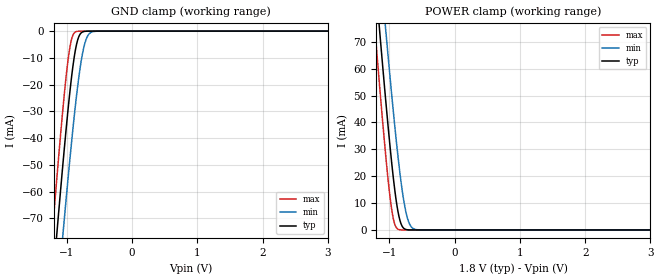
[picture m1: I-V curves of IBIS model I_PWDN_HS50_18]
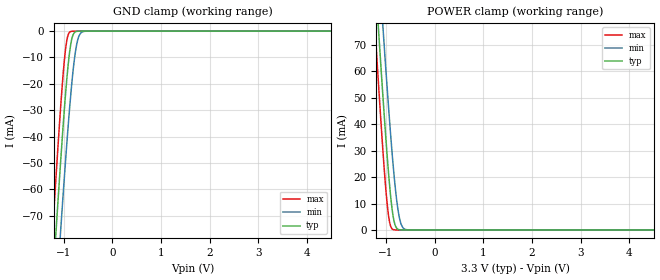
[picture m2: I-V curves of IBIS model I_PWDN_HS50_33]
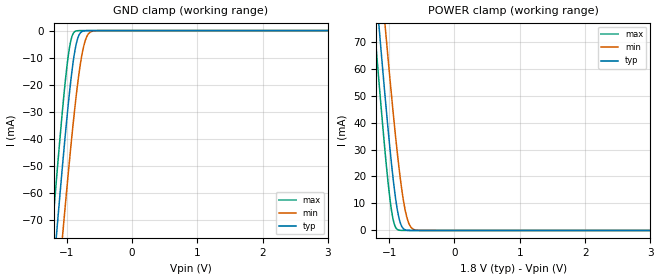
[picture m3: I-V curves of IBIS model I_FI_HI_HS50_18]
| Texas Instruments Incorporated
| DS90UB904Q
| 10-43-MHz 18-Bit Color FPD Link III Serializer and Deserializer
| with Bi-Directional Control Channel
| Marketing part#   Voltage Range   Package-type   Temperature
| DS90UB904QSQE   1.71V - 3.6V   48-Pin LLP   -40 to 105C
| DS90UB904QSQ   1.71V - 3.6V   48-Pin LLP   -40 to 105C
| DS90UB904QSQX   1.71V - 3.6V   48-Pin LLP   -40 to 105C
[IBIS Ver]   4.0
[File name]   ds90ub904q.ibs
[File Rev]   1.0
[Date]   04/11/2012
[Source]   Model built from TISPICE simulations at:
   Texas Instruments Incorporated.
   WEBENCH DESIGN CENTER
   12500 TI Blvd
   Dallas, TX -75243
   For Support e-mail: elab_scm_ibis@list.ti.com
[Notes]   Rev 1.0: 04/11/2012
   - Initial version of the IBIS model
   - All models are generated in Spectre
   - ccomp is listed in numerical order, for PVT information,
   please check notes above ccomp keyword for each model
   - All non-monotonic warnings can be ignored as per buffer behavior
[Disclaimer] This product is designed as an aid for customers of Texas Instruments.
   No warranties, either expressed or implied, with respect to this third
   party software (if any) or with respect to its fitness for any
   particular purpose is claimed by Texas Instruments or the author. The
   software (if any) is provided solely on an "as is" basis. The entire
   risk as to its quality and performance is with the customer
[Copyright]   (C)Copyright 2012 Texas Instruments Incorporated.
   All rights reserved.
|   DS90UB904Q
[Component]  DS90UB904Q
[Manufacturer]  Texas Instruments, Inc.
[Package]   |48-pin LLP 7.0x7.0x0.5mm
|   typ   min   max
R_pkg   0   0   0
L_pkg   0   0   0
C_pkg   0   0   0
[Pin]   signal_name   model_name   R_pin   L_pin   C_pin
1   SDA   IO_SMBUS_HS50
2   SCL   IO_SMBUS_HS50
3   VDDSSCG   POWER
4   PCLK   IO_CLK_50_HS50
5   ROUT[20]   IO_DATA_50_ATP_HS50
6   ROUT[19]   IO_DATA_50_HS50
7   VDDIO3   POWER
8   ROUT[18]   IO_DATA_50_HS50
9   ROUT[17]   IO_DATA_50_HS50
10   ROUT[16]   IO_DATA_50_HS50
11   ROUT[15]   IO_DATA_50_HS50
12   ROUT[14]   IO_DATA_50_HS50
13   ROUT[13]   IO_DATA_50_HS50
14   ROUT[12]   IO_DATA_50_HS50
15   ROUT[11]   IO_DATA_50_HS50
16   ROUT[10]   IO_DATA_50_HS50
17   VDDD   POWER
18   ROUT[9]   IO_DATA_50_HS50
19   ROUT[8]   IO_DATA_50_HS50
20   VDDIO2   POWER
21   ROUT[7]   IO_DATA_50_HS50
22   ROUT[6]   IO_DATA_50_HS50
23   ROUT[5]   IO_DATA_50_HS50
24   ROUT[4]   IO_DATA_50_HS50
25   ROUT[3]   IO_DATA_50_HS50
26   ROUT[2]   IO_DATA_50_HS50
27   ROUT[1]   IO_DATA_50_ATP_HS50
28   ROUT[0]   IO_DATA_50_ATP_HS50
29   VDDIO1   POWER
30   GPI[3]   IO_DATA_50_ATP_HS50
31   GPI[2]   IO_DATA_50_ATP_HS50
32   GPI[1]   IO_DATA_50_ATP_HS50
33   GPI[0]   IO_DATA_50_ATP_HS50
34   LOCK   IO_DATA_50_ATP_HS50
35   PDB   I_PWDN_HS50
36   VDDR   POWER
37   PASS   IO_DATA_50_HS50
38   RES   NC
39   RES   NC
40   VDDCML   POWER
41   RIN+   NC
42   RIN-   NC
43   RES   NC
44   BISTEN   I_PWDN_HS50
45   VDDPLL   POWER
46   RES   NC
47   MODE   I_FI_HI_HS50
48   ID[x]   NC
49   DAP   GND
[Package Model] llp48_ds90uh904
[Model Selector]   I_PWDN_HS50
I_PWDN_HS50_33   I_PWDN_HS50 input with VDD=3.3V
I_PWDN_HS50_18   I_PWDN_HS50 input with VDD=1.8V
[Model Selector]   I_FI_HI_HS50
I_FI_HI_HS50_33   I_FI_HI_HS50 input with VDD=3.3V
I_FI_HI_HS50_18   I_FI_HI_HS50 input with VDD=1.8V
[Model Selector]   IO_DATA_50_ATP_HS50
IO_DATA_50_ATP_HS50_33   IO_DATA_50_ATP_HS50 with VDD=3.3V
IO_DATA_50_ATP_HS50_18   IO_DATA_50_ATP_HS50 with VDD=1.8V
[Model Selector]   IO_DATA_50_HS50
IO_DATA_50_HS50_33   IO_DATA_50_HS50 with VDD=3.3V
IO_DATA_50_HS50_18   IO_DATA_50_HS50 with VDD=1.8V
[Model Selector]   IO_SMBUS_HS50
IO_SMBUS_HS50_33   IO_SMBUS_HS50 with VDD=3.3V
IO_SMBUS_HS50_18   IO_SMBUS_HS50 with VDD=1.8V
[Model Selector]   IO_CLK_50_HS50
IO_CLK_50_HS50_33   IO_CLK_50_HS50 with VDD=3.3V
IO_CLK_50_HS50_18   IO_CLK_50_HS50 with VDD=1.8V
|   Package model for DS90UB903
[Define Package Model]  llp48_ds90uh904
[Manufacturer]  Texas Instruments, Inc.
[OEM]  Texas Instruments, Inc.
[Description]  Package model with Au wires, simulation frequency of 1.4GHz
|Buildsheet# DS90UB904QSQ-03
[Number Of Pins]  48
[Pin Numbers]
49   | 49 = DAP
1   | 1 = L1
2   | 2 = L2
3   | 3 = L3
4   | 4 = L4
5   | 5 = L5
6   | 6 = L6
7   | 7 = L7
8   | 8 = L8
9   | 9 = L9
10   | 10 = L10
11   | 11 = L11
12   | 12 = L12
13   | 13 = L13
14   | 14 = L14
15   | 15 = L15
16   | 16 = L16
17   | 17 = L17
18   | 18 = L18
19   | 19 = L19
20   | 20 = L20
21   | 21 = L21
22   | 22 = L22
23   | 23 = L23
24   | 24 = L24
25   | 25 = L25
26   | 26 = L26
27   | 27 = L27
28   | 28 = L28
29   | 29 = L29
30   | 30 = L30
31   | 31 = L31
32   | 32 = L32
33   | 33 = L33
34   | 34 = L34
35   | 35 = L35
36   | 36 = L36
37   | 37 = L37
38   | 38 = L38
39   | 39 = L39
40   | 40 = L40
41   | 41 = L41
42   | 42 = L42
44   | 44 = L44
45   | 45 = L45
46   | 46 = L46
47   | 47 = L47
48   | 48 = L48
[Model Data]
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[End Model Data]
[End Package Model]
| Models and submodels in the file (12): I_PWDN_HS50_18 (Input), I_PWDN_HS50_33 (Input), I_FI_HI_HS50_18 (Input), I_FI_HI_HS50_33 (Input), IO_DATA_50_ATP_HS50_33 (I/O), IO_DATA_50_ATP_HS50_18 (I/O), IO_DATA_50_HS50_33 (I/O), IO_DATA_50_HS50_18 (I/O), IO_SMBUS_HS50_33 (I/O_open_drain), IO_SMBUS_HS50_18 (I/O_open_drain), IO_CLK_50_HS50_33 (I/O), IO_CLK_50_HS50_18 (I/O)
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|   Model I_PWDN_HS50_18
[Model]   I_PWDN_HS50_18
Model_type   Input
Vinl = 0.63V
Vinh = 1.17V
|   typ   min   max
|   (nom)   (weak)   (fast)
C_comp   0.5928pF   0.5928pF   0.5928pF
[Voltage Range]   1.800V   1.710V   1.890V
[Temperature Range]   25.0   105.0   -40.0
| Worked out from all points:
|   GND clamp passes 1 mA (typ) near -0.79 V on its own axis
|   POWER clamp passes 1 mA (typ) near -0.79 V on its own axis
[GND Clamp]
|   Voltage   I(typ)   I(min)   I(max)
-1.8V     -270.9mA   -291mA     -255.6mA
-1.228V   -97.1mA    -122.7mA   -76.77mA
-1.201V   -89.21mA   -115mA     -68.71mA
-1.147V   -73.63mA   -99.73mA   -52.87mA
-1.055V   -48.06mA   -74.39mA   -27.51mA
-957.6mV  -23.54mA   -48.82mA   -6.663mA
-871.2mV  -7.328mA   -28.21mA   -335.2uA
-811.8mV  -1.781mA   -16.28mA   -25.67uA
-741.6mV  -161.6uA   -6.205mA   -6.921uA
-682.2mV  -20.1uA    -1.83mA    -5.854uA
-601.2mV  -4.02uA    -199.2uA   -5.127uA
3.595V    6.712uA    3.483uA    12.03uA
[POWER Clamp]
|   Voltage   I(typ)   I(min)   I(max)
-1.8V     270.2mA    290.2mA    254.8mA
-1.228V   96.77mA    122.3mA    76.49mA
-1.201V   88.9mA     114.6mA    68.45mA
-1.147V   73.36mA    99.39mA    52.65mA
-1.055V   47.86mA    74.11mA    27.37mA
-957.6mV  23.41mA    48.61mA    6.6mA
-871.2mV  7.262mA    28.06mA    325.8uA
-811.8mV  1.758mA    16.17mA    20.65uA
-741.6mV  156.5uA    6.146mA    2.661uA
-682.2mV  17.07uA    1.807mA    2.011uA
-601.2mV  1.608uA    195uA      1.824uA
3.595V    0A         0A         0A
|   Model I_PWDN_HS50_33
[Model]   I_PWDN_HS50_33
Model_type   Input
Vinl = 0.8V
Vinh = 2.0V
|   typ   min   max
|   (nom)   (weak)   (fast)
C_comp   0.5928pF   0.5928pF   0.5928pF
[Voltage Range]   3.300V   3.000V   3.600V
[Temperature Range]   25.0   105.0   -40.0
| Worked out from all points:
|   GND clamp passes 1 mA (typ) near -0.79 V on its own axis
|   POWER clamp passes 1 mA (typ) near -0.79 V on its own axis
[GND Clamp]
|   Voltage   I(typ)   I(min)   I(max)
-3.3V     -740.6mA   -745.8mA   -738.2mA
-1.231V   -98.06mA   -123.6mA   -77.76mA
-1.221V   -95.16mA   -120.8mA   -74.79mA
-1.171V   -80.77mA   -106.7mA   -60.12mA
-1.142V   -72.26mA   -98.38mA   -51.49mA
-1.063V   -50.17mA   -76.5mA    -29.54mA
-953.7mV  -22.65mA   -47.84mA   -6.095mA
-914.1mV  -14.38mA   -38.09mA   -1.938mA
-854.7mV  -5.279mA   -24.66mA   -158.3uA
-735.9mV  -131.2uA   -5.62mA    -6.724uA
-597.3mV  -3.893uA   -177.7uA   -5.09uA
6.59V     7.865uA    3.955uA    14.61uA
[POWER Clamp]
|   Voltage   I(typ)   I(min)   I(max)
-3.3V     739mA      744.2mA    736.5mA
-1.231V   97.8mA     123.3mA    77.52mA
-1.221V   94.9mA     120.5mA    74.56mA
-1.171V   80.54mA    106.4mA    59.92mA
-1.142V   72.04mA    98.11mA    51.31mA
-1.063V   50mA       76.28mA    29.42mA
-953.7mV  22.55mA    47.67mA    6.048mA
-914.1mV  14.3mA     37.95mA    1.916mA
-854.7mV  5.24mA     24.55mA    149.8uA
-735.9mV  126.1uA    5.58mA     498.8nA
-597.3mV  637nA      174.2uA    50.05nA
6.59V     0A         0A         0A
|   I_FI_HI_HS50_18   Input model
[Model]   I_FI_HI_HS50_18
Model_type   Input
Vinl = 0.63V
Vinh = 1.17V
|   typ   min   max
|   (nom)   (weak)   (strong)
C_comp   0.6368pF   0.6368pF   0.6368pF
[Voltage Range]   1.800V   1.710V   1.890V
[Temperature Range]   25.0   105.0   -40.0
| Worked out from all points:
|   GND clamp passes 1 mA (typ) near -0.79 V on its own axis
|   POWER clamp passes 1 mA (typ) near -0.79 V on its own axis
[GND Clamp]
|   Voltage   I(typ)   I(min)   I(max)
-1.8V     -270.3mA   -290.3mA   -255mA
-1.228V   -96.82mA   -122.3mA   -76.53mA
-1.201V   -88.95mA   -114.7mA   -68.49mA
-1.147V   -73.41mA   -99.45mA   -52.69mA
-1.055V   -47.89mA   -74.16mA   -27.39mA
-957.6mV  -23.43mA   -48.64mA   -6.613mA
-871.2mV  -7.275mA   -28.08mA   -326.1uA
-811.8mV  -1.763mA   -16.19mA   -19.76uA
-741.6mV  -156.8uA   -6.157mA   -1.787uA
-682.2mV  -16.95uA   -1.812mA   -1.235uA
-601.2mV  -1.489uA   -195.7uA   -1.204uA
3.595V    0A         0A         0A
[POWER Clamp]
|   Voltage   I(typ)   I(min)   I(max)
-1.8V     270.3mA    290.4mA    255mA
-1.228V   96.84mA    122.3mA    76.55mA
-1.201V   88.97mA    114.7mA    68.51mA
-1.147V   73.43mA    99.47mA    52.71mA
-1.055V   47.91mA    74.18mA    27.41mA
-957.6mV  23.45mA    48.67mA    6.633mA
-871.2mV  7.3mA      28.11mA    334.5uA
-811.8mV  1.784mA    16.22mA    21.24uA
-741.6mV  164.9uA    6.189mA    2.38uA
-682.2mV  18.56uA    1.84mA     1.645uA
-601.2mV  1.748uA    209.3uA    1.397uA
3.595V    0A         0A         0A
